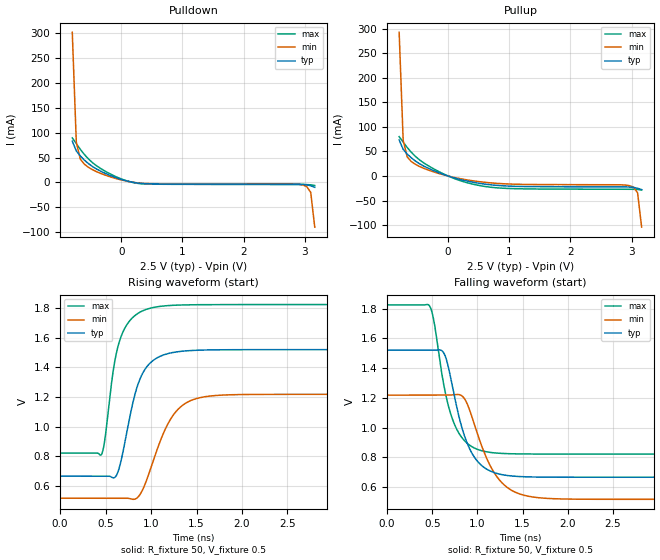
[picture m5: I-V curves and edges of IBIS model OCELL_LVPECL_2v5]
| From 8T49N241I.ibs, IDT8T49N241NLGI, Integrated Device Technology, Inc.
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| 4.00000e+00   -1.40218e-02   -7.79461e-01   -2.57100e-03
| 4.10000e+00   -3.15780e-02   -1.61164e+00   -1.15565e-02
| 4.20000e+00   -2.42978e-01   -2.44445e+00   -2.65858e-02
| 4.30000e+00   -1.11769e+00   -3.27769e+00   -4.22799e-02
| 4.40000e+00   -2.23090e+00   -4.11128e+00   -8.93843e-02
| 4.50000e+00   -3.34464e+00   -4.94518e+00   -8.46638e-01
| 4.60000e+00   -4.45885e+00   -5.77938e+00   -2.27113e+00
| 4.70000e+00   -5.57349e+00   -6.61386e+00   -3.69616e+00
| 4.80000e+00   -6.68850e+00   -7.44861e+00   -5.12164e+00
| 4.90000e+00   -7.80386e+00   -8.28360e+00   -6.54748e+00
| 5.00000e+00   -8.91950e+00   -9.11883e+00   -7.97363e+00
| 5.10000e+00   -1.00354e+01   -9.95428e+00   -9.40002e+00
| 5.20000e+00   -1.11515e+01   -1.07899e+01   -1.08266e+01
| 5.30000e+00   -1.22678e+01   -1.16258e+01   -1.22534e+01
| 5.40000e+00   -1.33842e+01   -1.24618e+01   -1.36803e+01
| 5.50000e+00   -1.45008e+01   -1.32980e+01   -1.51073e+01
| 5.60000e+00   -1.56175e+01   -1.41343e+01   -1.65344e+01
| 5.70000e+00   -1.67343e+01   -1.49707e+01   -1.79616e+01
| 5.80000e+00   -1.78512e+01   -1.58073e+01   -1.93888e+01
| 5.90000e+00   -1.89682e+01   -1.66440e+01   -2.08161e+01
| 6.00000e+00   -2.00852e+01   -1.74808e+01   -2.22434e+01
| 6.10000e+00   -2.12022e+01   -1.83178e+01   -2.36707e+01
| 6.20000e+00   -2.23193e+01   -1.91548e+01   -2.50980e+01
| 6.30000e+00   -2.34365e+01   -1.99919e+01   -2.65253e+01
| 6.40000e+00   -2.45536e+01   -2.08290e+01   -2.79526e+01
| 6.50000e+00   -2.56708e+01   -2.16663e+01   -2.93798e+01
| 6.60000e+00   -2.67880e+01   -2.25036e+01   -3.08071e+01
[Model] OCELL_LVPECL_2v5
Model_type   Output_ECL
Polarity   Non-Inverting
|   typ   min   max
C_comp   2pF   1.5pF   2.5pF
Vmeas = 1.112V
Rref = 50
Cref = 0
Vref = 0.5V
|   typ   min   max
[Voltage range]   2.5V   2.375V   2.625V
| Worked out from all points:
|   rising waveform, R_fixture 50, V_fixture 0.5: 20-80 % time 205ps typ, 282ps min, 166ps max; typ from 0.666 V to 1.52 V
|   falling waveform, R_fixture 50, V_fixture 0.5: 20-80 % time 232ps typ, 294ps min, 202ps max; typ from 1.52 V to 0.666 V
[Pulldown]
|Voltage   I (typ)   I (min)   I (max)
|Note, modeling breaks down at 250mA and above.  This is well beyond the functional   |
|operating range of the device.  Should this scenario occur, catastrophic failure and   |
|possible damage to the device and/or board is of higher concern than the I-V curve   |
|behavior.  The IBIS checker will flag currents in excess of 10A with warnings.  Lines   |
|with currents in excess of 0.35 A have been commented out.  The points still remain|
|available to the user if the user desires to use them.   |
|-2.20000e+00   3.02004e+01   2.66706e+01   3.62378e+01
|-1.90000e+00   2.33363e+01   2.09561e+01   2.74628e+01
|-1.60000e+00   1.64758e+01   1.52450e+01   1.86917e+01
|-1.30000e+00   9.61893e+00   9.53719e+00   9.92462e+00
|-1.00000e+00   2.76578e+00   3.83258e+00   1.16404e+00
|-9.99000e-01   2.74294e+00   3.81357e+00   1.13587e+00
|-9.32920e-01   1.23395e+00   2.55739e+00   1.61783e-01
|-8.66839e-01   2.16574e-01   1.30123e+00   1.00510e-01
-800.8mV  82.79mA    301.1mA    89.39mA
-734.7mV  63.32mA    80.64mA    78.02mA
-668.6mV  53.13mA    46.51mA    66.36mA
-602.5mV  44.88mA    36.56mA    56.09mA
-404.3mV  27.04mA    21.73mA    33.53mA
-206mV    15.41mA    12.43mA    18.81mA
58.29mV   4.159mA    3.498mA    4.603mA
256.5mV   -922.3uA   -616.9uA   -1.508mA
2.966V    -3.758mA   -4.886mA   -4.158mA
3.032V    -4.613mA   -8.064mA   -4.232mA
3.098V    -6.517mA   -19.72mA   -4.645mA
3.164V    -9.585mA   -89.55mA   -6.094mA
| 3.23015e+00   -1.39486e-02   -5.08117e-01   -9.17103e-03
| 3.29623e+00   -2.26187e-02   -1.11809e+00   -1.38071e-02
| 3.36231e+00   -7.55282e-02   -1.72828e+00   -1.96181e-02
| 3.42839e+00   -5.32427e-01   -2.33864e+00   -2.58190e-02
| 3.49447e+00   -1.26543e+00   -2.94912e+00   -3.27151e-02
| 3.56055e+00   -1.99865e+00   -3.55972e+00   -6.64489e-02
| 3.62663e+00   -2.73208e+00   -4.17042e+00   -5.72680e-01
| 3.69271e+00   -3.46570e+00   -4.78120e+00   -1.51037e+00
| 3.75879e+00   -4.19950e+00   -5.39207e+00   -2.44820e+00
| 3.82487e+00   -4.93344e+00   -6.00302e+00   -3.38614e+00
| 3.89095e+00   -5.66751e+00   -6.61405e+00   -4.32416e+00
| 3.95703e+00   -6.40169e+00   -7.22514e+00   -5.26226e+00
| 4.02311e+00   -7.13596e+00   -7.83630e+00   -6.20045e+00
| 4.08920e+00   -7.87031e+00   -8.44752e+00   -7.13878e+00
| 4.15528e+00   -8.60474e+00   -9.05881e+00   -8.07728e+00
| 4.22136e+00   -9.33924e+00   -9.67015e+00   -9.01596e+00
| 4.28744e+00   -1.00738e+01   -1.02815e+01   -9.95479e+00
| 4.35352e+00   -1.08084e+01   -1.08930e+01   -1.08937e+01
| 4.41960e+00   -1.15431e+01   -1.15045e+01   -1.18328e+01
| 4.48568e+00   -1.22778e+01   -1.21160e+01   -1.27719e+01
| 4.55176e+00   -1.30125e+01   -1.27276e+01   -1.37110e+01
| 4.61784e+00   -1.37473e+01   -1.33392e+01   -1.46502e+01
| 4.68392e+00   -1.44822e+01   -1.39509e+01   -1.55895e+01
| 4.75000e+00   -1.52170e+01   -1.45626e+01   -1.65287e+01
| 4.75100e+00   -1.52281e+01   -1.45718e+01   -1.65429e+01
| 4.80080e+00   -1.57820e+01   -1.50328e+01   -1.72508e+01
| 4.85060e+00   -1.63358e+01   -1.54939e+01   -1.79587e+01
| 4.90040e+00   -1.68897e+01   -1.59549e+01   -1.86666e+01
| 4.95020e+00   -1.74436e+01   -1.64160e+01   -1.93745e+01
| 5.00000e+00   -1.79975e+01   -1.68771e+01   -2.00824e+01
[Pullup]
|Voltage   I (typ)   I (min)   I (max)
|Note, modeling breaks down at 250mA and above.  This is well beyond the functional   |
|operating range of the device.  Should this scenario occur, catastrophic failure and   |
|possible damage to the device and/or board is of higher concern than the I-V curve   |
|behavior.  The IBIS checker will flag currents in excess of 10A with warnings.  Lines   |
|with currents in excess of 0.35 A have been commented out.  The points still remain|
|available to the user if the user desires to use them.   |
|-2.20000e+00   3.02143e+01   2.66849e+01   3.62508e+01
|-1.90000e+00   2.33430e+01   2.09644e+01   2.74692e+01
|-1.60000e+00   1.64760e+01   1.52468e+01   1.86950e+01
|-1.30000e+00   9.61479e+00   9.53307e+00   9.92303e+00
|-1.00000e+00   2.75802e+00   3.82494e+00   1.15737e+00
|-9.99000e-01   2.73517e+00   3.80592e+00   1.12918e+00
|-9.32920e-01   1.22549e+00   2.54926e+00   1.54070e-01
|-8.66839e-01   2.07498e-01   1.29270e+00   9.18618e-02
-800.8mV  73.34mA    292.4mA    80.08mA
-734.7mV  54.19mA    72.32mA    68.89mA
-668.6mV  44.7mA     38.83mA    57.96mA
-602.5mV  37.09mA    29.48mA    48.38mA
-404.3mV  20.56mA    15.9mA     27.09mA
-73.87mV  3.148mA    2.402mA    4.206mA
586.9mV   -16.24mA   -12.6mA    -20.98mA
1.182V    -21.25mA   -16.94mA   -26.01mA
2.966V    -22.42mA   -19.65mA   -26.96mA
3.032V    -23.22mA   -22.69mA   -27.03mA
3.098V    -24.99mA   -34.25mA   -27.37mA
3.164V    -27.75mA   -104.1mA   -28.72mA
| 3.23015e+00   -3.17112e-02   -5.22679e-01   -3.15890e-02
| 3.29623e+00   -3.99976e-02   -1.13270e+00   -3.58009e-02
| 3.36231e+00   -9.26644e-02   -1.74295e+00   -4.10841e-02
| 3.42839e+00   -5.49519e-01   -2.35335e+00   -4.67634e-02
| 3.49447e+00   -1.28265e+00   -2.96387e+00   -5.31907e-02
| 3.56055e+00   -2.01607e+00   -3.57450e+00   -8.64790e-02
| 3.62663e+00   -2.74972e+00   -4.18523e+00   -5.92271e-01
| 3.69271e+00   -3.48355e+00   -4.79604e+00   -1.52958e+00
| 3.75879e+00   -4.21751e+00   -5.40693e+00   -2.46723e+00
| 3.82487e+00   -4.95159e+00   -6.01789e+00   -3.40527e+00
| 3.89095e+00   -5.68576e+00   -6.62893e+00   -4.34358e+00
| 3.95703e+00   -6.42002e+00   -7.24004e+00   -5.28210e+00
| 4.02311e+00   -7.15435e+00   -7.85122e+00   -6.22081e+00
| 4.08920e+00   -7.88876e+00   -8.46245e+00   -7.15965e+00
| 4.15528e+00   -8.62323e+00   -9.07375e+00   -8.09859e+00
| 4.22136e+00   -9.35777e+00   -9.68511e+00   -9.03761e+00
| 4.28744e+00   -1.00924e+01   -1.02965e+01   -9.97668e+00
| 4.35352e+00   -1.08270e+01   -1.09080e+01   -1.09158e+01
| 4.41960e+00   -1.15617e+01   -1.15195e+01   -1.18550e+01
| 4.48568e+00   -1.22964e+01   -1.21310e+01   -1.27942e+01
| 4.55176e+00   -1.30312e+01   -1.27426e+01   -1.37334e+01
| 4.61784e+00   -1.37660e+01   -1.33543e+01   -1.46727e+01
| 4.68392e+00   -1.45009e+01   -1.39660e+01   -1.56120e+01
| 4.75000e+00   -1.52358e+01   -1.45777e+01   -1.65513e+01
| 4.75100e+00   -1.52469e+01   -1.45869e+01   -1.65655e+01
| 4.80080e+00   -1.58008e+01   -1.50480e+01   -1.72734e+01
| 4.85060e+00   -1.63546e+01   -1.55090e+01   -1.79814e+01
| 4.90040e+00   -1.69085e+01   -1.59701e+01   -1.86893e+01
| 4.95020e+00   -1.74625e+01   -1.64312e+01   -1.93973e+01
| 5.00000e+00   -1.80164e+01   -1.68923e+01   -2.01052e+01
[Ramp]
|   typ   min   max
dV/dt_r   0.519/0.206n   0.425/0.283n   0.61/0.166n
dV/dt_f   0.514/0.231n   0.423/0.294n   0.604/0.202n
R_load =   50.0000
[Rising Waveform]
R_fixture = 50
V_fixture = 0.5   | VCC_typ - 2V
V_fixture_max = 0.625   | VCC_max - 2V
V_fixture_min = 0.375   | VCC_min - 2V
C_fixture = 0.0p
| Time   typ   min   max
0s        665.9mV    517.2mV    822mV
457.8ps   665.9mV    517.2mV    816.4mV
493.3ps   665.9mV    517.2mV    920.5mV
586.7ps   654.8mV    517.2mV    1.39V
644.4ps   711mV      517.2mV    1.561V
813.3ps   1.196V     510mV      1.746V
920ps     1.375V     591.7mV    1.786V
1.2ns     1.496V     1.036V     1.818V
1.476ns   1.516V     1.186V     1.824V
4ns       1.521V     1.219V     1.825V
[Falling Waveform]
R_fixture = 50
V_fixture = 0.5   | VCC_typ - 2V
V_fixture_max = 0.625   | VCC_max - 2V
V_fixture_min = 0.375   | VCC_min - 2V
C_fixture = 0.0p
| Time   typ   min   max
0s        1.521V     1.218V     1.826V
471.1ps   1.521V     1.218V     1.819V
520ps     1.521V     1.218V     1.713V
622.2ps   1.508V     1.218V     1.306V
711.1ps   1.315V     1.22V      1.08V
853.3ps   950.4mV    1.198V     914.2mV
991.1ps   780.7mV    975.3mV    855.8mV
1.222ns   690.3mV    663.9mV    828.1mV
1.524ns   669mV      543.2mV    822.5mV
4ns       665.9mV    517.2mV    821.9mV
